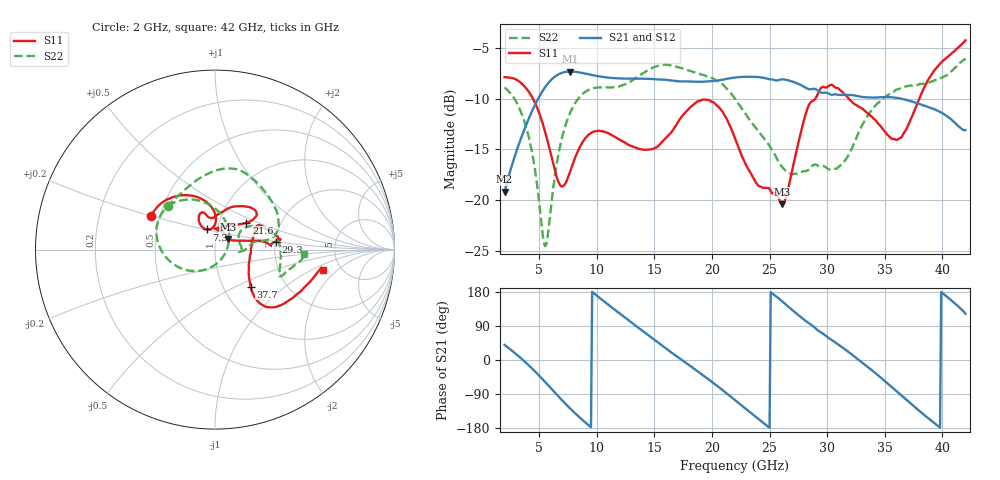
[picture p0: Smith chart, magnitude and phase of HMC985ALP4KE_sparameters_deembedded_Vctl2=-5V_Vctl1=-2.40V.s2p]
!s2p File: Measurements: S11, S21, S12, S22
# GHz S dB R 50.0
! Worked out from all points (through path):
!   401 points, 2 GHz to 42 GHz, reference 50 ohm
!   highest |S21| = -7.34 dB at 7.7 GHz (marker M1); lowest = -19.2 dB at 2 GHz (marker M2)
!   lowest |S11| = -20.4 dB at 26.1 GHz (marker M3), VSWR 1.21, Z = 57.7 + j6.91 ohm
!   |S11| at or under -10 dB: 4.459 GHz to 28.98 GHz (24.52 GHz wide, 147 % of centre); 31.87 GHz to 38 GHz (6.129 GHz wide, 17.5 % of centre)
!   |S22| runs from -24.5 to -6.0 dB; largest |S21 - S12| = 0.00054
!   S11 on the Smith chart (normalised r, x): 2 GHz: 0.45, +0.20; 7.3 GHz: 0.89, +0.20; 21.6 GHz: 1.35, +0.42; 29.3 GHz: 2.02, +0.21; 37.7 GHz: 1.34, -0.60; 42 GHz: 3.63, -1.31
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2  -7.89 152.3  -19.16 39.8  -19.17 39.8  -8.91 137.2
4  -9.18 119.2  -12.23 -11.2  -12.23 -11.2  -13.36 85.4
5.5  -13.21 92.0  -8.90 -57.3  -8.90 -57.3  -24.52 -25.9
6.6  -17.98 94.1  -7.66 -93.7  -7.66 -93.7  -15.91 -131.4
7.3  -18.30 112.4  -7.37 -116.1  -7.38 -116.1  -12.57 -157.4
7.7  -17.14 118.6  -7.34 -128.3  -7.34 -128.3  -11.37 -169.1
8.7  -14.42 118.5  -7.47 -156.7  -7.47 -156.7  -9.62 168.4
10.3  -13.19 109.1  -7.83 162.6  -7.84 162.7  -8.90 145.0
12.3  -14.23 103.4  -8.03 115.5  -8.03 115.5  -8.67 120.2
15.4  -14.61 88.9  -8.13 44.1  -8.14 44.1  -6.76 80.1
18.3  -10.68 55.5  -8.34 -19.8  -8.34 -19.7  -7.35 51.1
21.6  -12.78 40.5  -8.00 -96.0  -8.01 -95.9  -9.41 12.8
22  -13.87 44.7  -7.92 -105.9  -7.93 -105.8  -10.01 11.1
24.1  -18.62 86.8  -7.89 -157.1  -7.90 -157.0  -13.34 10.3
26.1  -20.39 38.4  -8.11 154.8  -8.11 154.8  -16.74 -3.7
28.7  -10.23 4.4  -9.06 91.1  -9.07 91.2  -16.62 0.4
29.3  -9.26 7.5  -9.31 76.0  -9.31 76.1  -16.65 2.9
32.5  -10.61 26.0  -9.72 5.9  -9.73 6.0  -13.97 36.1
35.4  -13.73 6.6  -9.86 -65.9  -9.86 -65.8  -9.56 15.2
37.7  -10.86 -46.2  -10.40 -126.4  -10.41 -126.3  -8.64 -6.1
39.7  -6.69 -43.8  -11.25 -175.9  -11.25 -175.9  -8.08 -22.4
42  -4.28 -10.6  -13.10 122.2  -13.11 122.2  -6.04 -3.1
